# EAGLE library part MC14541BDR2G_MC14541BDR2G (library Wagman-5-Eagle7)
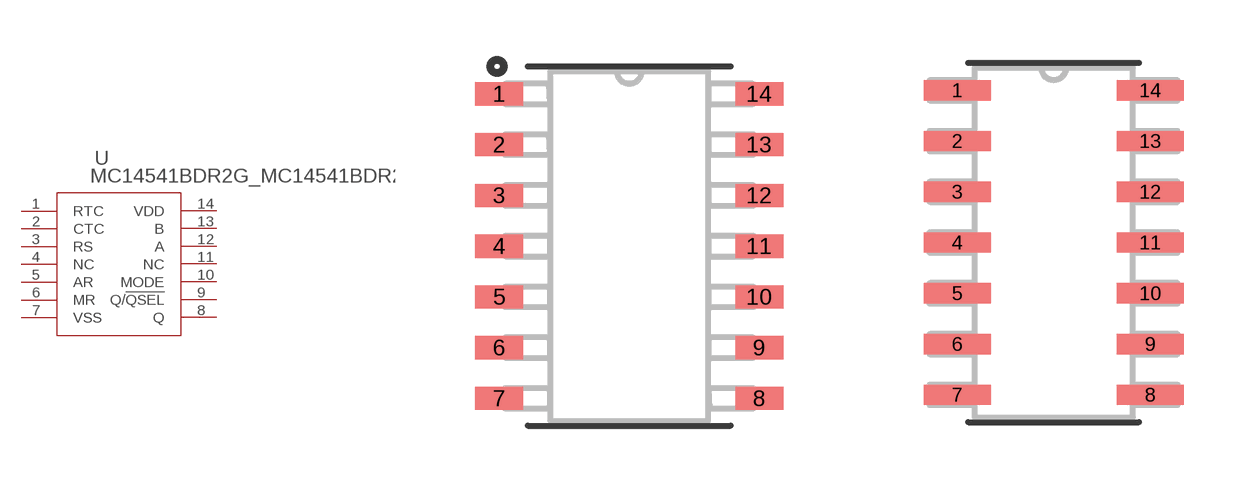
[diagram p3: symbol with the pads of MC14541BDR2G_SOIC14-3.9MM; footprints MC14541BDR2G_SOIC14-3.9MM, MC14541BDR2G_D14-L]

Designator prefix U

## MC14541BDR2G_MC14541BDR2G (MANUFACTURER_PART_NUMBER: SN74HCT74DR; VENDOR: Vendor)  [MC14541BDR2G_SOIC14-3.9MM]
1  RTC  in
2  CTC  in
3  RS  in
4  NC  in
5  AR  out
6  MR  out
7  VSS  pwr
8  Q  out
9  Q/!QSEL  out
10  MODE  in
11  NC  in
12  A  in
13  B  in
14  VDD  pwr

## MC14541BDR2G_MC14541BDR2GD14-L (MANUFACTURER_PART_NUMBER: SN74HCT74DR; VENDOR: Vendor)  [MC14541BDR2G_D14-L]
Pads as for MC14541BDR2G_SOIC14-3.9MM

## MC14541BDR2G_MC14541BDR2GD14-M (MANUFACTURER_PART_NUMBER: SN74HCT74DR; VENDOR: Vendor)  [MC14541BDR2G_D14-M]
Pads as for MC14541BDR2G_SOIC14-3.9MM

## Footprint MC14541BDR2G_SOIC14-3.9MM (pad centres in mm)
smd 1.2 x 0.58: 1 -3.25,3.81; 2 -3.25,2.54; 3 -3.25,1.27; 4 -3.25,0; 5 -3.25,-1.27; 6 -3.25,-2.54; 7 -3.25,-3.81; 8 3.25,-3.81; 9 3.25,-2.54; 10 3.25,-1.27; 11 3.25,0; 12 3.25,1.27; 13 3.25,2.54; 14 3.25,3.81

## Footprint MC14541BDR2G_D14-L (pad centres in mm)
smd 1.676 x 0.508: 1 -2.413,3.81; 2 -2.413,2.54; 3 -2.413,1.27; 4 -2.413,0; 5 -2.413,-1.27; 6 -2.413,-2.54; 7 -2.413,-3.81; 8 2.413,-3.81; 9 2.413,-2.54; 10 2.413,-1.27; 11 2.413,0; 12 2.413,1.27; 13 2.413,2.54; 14 2.413,3.81

## Footprint MC14541BDR2G_D14-M (pad centres in mm)
smd 2.286 x 0.61: 1 -2.515,3.81; 2 -2.515,2.54; 3 -2.515,1.27; 4 -2.515,0; 5 -2.515,-1.27; 6 -2.515,-2.54; 7 -2.515,-3.81; 8 2.515,-3.81; 9 2.515,-2.54; 10 2.515,-1.27; 11 2.515,0; 12 2.515,1.27; 13 2.515,2.54; 14 2.515,3.81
